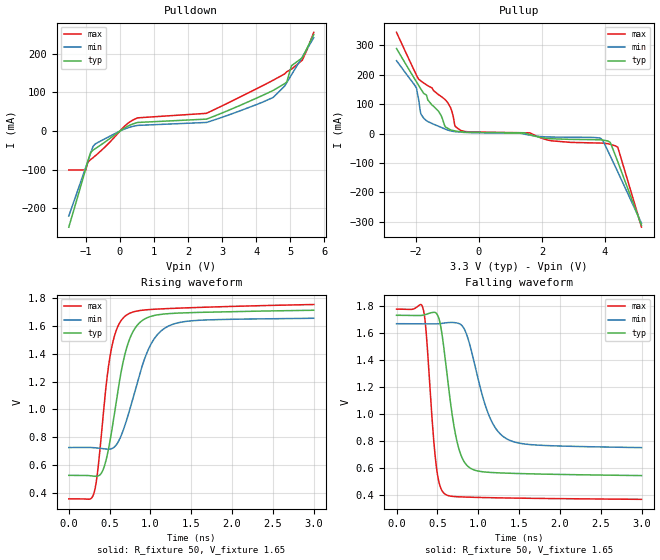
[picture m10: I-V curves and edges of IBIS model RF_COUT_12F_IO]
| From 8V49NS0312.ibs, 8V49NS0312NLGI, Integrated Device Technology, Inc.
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[Model]   RF_COUT_12F_IO
Model_type   Output
Polarity   Non-Inverting
|   typ   min   max
C_comp   2pF   1.5pF   2.5pF
Vmeas = 1.65V
Rref = 50
Cref = 0
Vref = 1.65V
|   typ   min   max
[Voltage range]   3.3V   3.135V   3.465V
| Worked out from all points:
|   slope of the pulldown table from 0 to 0.495 V, typ, clamps not added: 22.8 ohm
|   slope of the pullup table from 0 to 0.495 V, typ, clamps not added: 679 ohm
|   rising waveform, R_fixture 50, V_fixture 1.65: 20-80 % time 224ps typ, 305ps min, 167ps max; typ from 0.527 V to 1.71 V
|   falling waveform, R_fixture 50, V_fixture 1.65: 20-80 % time 167ps typ, 264ps min, 103ps max; typ from 1.73 V to 0.544 V
[Pulldown]
|Voltage   I (typ)   I (min)   I (max)
|Note, modeling breaks down at 250mA and above.  This is well beyond the functional   |
|operating range of the device.  Should this scenario occur, catastrophic failure and   |
|possible damage to the device and/or board is of higher concern than the I-V curve   |
|behavior.  The IBIS checker will flag currents in excess of 10A with warnings.  Lines   |
|with currents in excess of 0.35 A have been commented out.  The points still remain|
|available to the user if the user desires to use them.   |
|-3.30000e+00   -7.87257e-01   -6.73606e-01   -1.00473e-01
|-2.76540e+00   -6.25752e-01   -5.37099e-01   -1.00473e-01
|-2.74560e+00   -6.19818e-01   -5.32094e-01   -1.00473e-01
|-2.15160e+00   -4.42770e-01   -3.82988e-01   -1.00473e-01
|-1.97340e+00   -3.89863e-01   -3.38493e-01   -1.00473e-01
-1.498V   -248.5mA   -219.7mA   -100.5mA
-1V       -97.34mA   -93.55mA   -100.5mA
-943.8mV  -79.97mA   -79.2mA    -81.69mA
-787.2mV  -49.36mA   -39.79mA   -68.73mA
145.2mV   8.539mA    5.651mA    13.34mA
520mV     22.39mA    14.82mA    34.33mA
2.541V    31.09mA    22.47mA    46.04mA
4.462V    103.7mA    85.76mA    130mA
4.898V    127.4mA    125.6mA    153.7mA
5.034V    169.2mA    145.7mA    160.2mA
5.354V    190mA      192mA      183.8mA
5.689V    249.9mA    241.9mA    255.7mA
| 6.20400e+00   3.44362e-01   3.20728e-01   3.75765e-01
| 6.20480e+00   3.44511e-01   3.20853e-01   3.75955e-01
| 6.53920e+00   4.07706e-01   3.73926e-01   4.56273e-01
| 6.58480e+00   4.16452e-01   3.81302e-01   4.67382e-01
| 6.60000e+00   4.19374e-01   3.83769e-01   4.71095e-01
[Pullup]
|Voltage   I (typ)   I (min)   I (max)
|Note, modeling breaks down at 250mA and above.  This is well beyond the functional   |
|operating range of the device.  Should this scenario occur, catastrophic failure and   |
|possible damage to the device and/or board is of higher concern than the I-V curve   |
|behavior.  The IBIS checker will flag currents in excess of 10A with warnings.  Lines   |
|with currents in excess of 0.35 A have been commented out.  The points still remain|
|available to the user if the user desires to use them.   |
|-3.30000e+00   4.19294e-01   3.53041e-01   5.11558e-01
|-3.12180e+00   3.85262e-01   3.25457e-01   4.67756e-01
|-3.10200e+00   3.81510e-01   3.22421e-01   4.62928e-01
|-2.90400e+00   3.44298e-01   2.92352e-01   4.15047e-01
|-2.86440e+00   3.36919e-01   2.86398e-01   4.05555e-01
|-2.70600e+00   3.07607e-01   2.62761e-01   3.67856e-01
-2.607V   289.4mA    248.1mA    344.5mA
-1.973V   175.8mA    155.1mA    198.5mA
-1.835V   151.6mA    66.9mA     179.1mA
-1.736V   136.3mA    51.5mA     171.6mA
-1.063V   23.31mA    15.5mA     115.1mA
-884.4mV  12.55mA    9.074mA    85.79mA
-745.8mV  9.119mA    6.838mA    24.75mA
-567.6mV  6.452mA    5.027mA    10.81mA
3.848V    -20.97mA   -14.74mA   -31.9mA
4.165V    -29.65mA   -75.72mA   -36.12mA
4.402V    -95.36mA   -129.9mA   -45.91mA
5.155V    -312mA     -304.8mA   -317.9mA
| 5.29320e+00   -3.52204e-01   -3.37369e-01   -3.68931e-01
| 5.31300e+00   -3.57949e-01   -3.42027e-01   -3.76222e-01
| 5.41200e+00   -3.86685e-01   -3.65343e-01   -4.12676e-01
| 5.57040e+00   -4.32707e-01   -4.02726e-01   -4.71000e-01
| 5.66940e+00   -4.61500e-01   -4.26140e-01   -5.07454e-01
| 5.94660e+00   -5.42257e-01   -4.91910e-01   -6.09564e-01
| 5.98620e+00   -5.53812e-01   -5.01333e-01   -6.24160e-01
| 6.12480e+00   -5.94300e-01   -5.34374e-01   -6.75269e-01
| 6.14460e+00   -6.00090e-01   -5.39102e-01   -6.82574e-01
| 6.36240e+00   -6.63895e-01   -5.91253e-01   -7.63012e-01
| 6.38220e+00   -6.69707e-01   -5.96008e-01   -7.70333e-01
| 6.58020e+00   -7.27952e-01   -6.43704e-01   -8.43649e-01
| 6.60000e+00   -7.33790e-01   -6.48489e-01   -8.50992e-01
[Ramp]
|   typ   min   max
dV/dt_r   0.714/0.225n   0.563/0.307n   0.838/0.167n
dV/dt_f   0.727/0.169n   0.557/0.265n   0.867/0.105n
R_load =   50.0000
[Rising Waveform]
R_fixture = 50
V_fixture = 1.65   |Vcc_typ
V_fixture_min = 1.525  |Vcc_min
V_fixture_max = 1.7325 |Vcc_max
C_fixture = 0.0p
| Time   typ   min   max
0s        526.9mV    726.6mV    358.5mV
309.3ps   520.7mV    725.4mV    400.9mV
351.4ps   521.4mV    723.1mV    543.7mV
417.4ps   563mV      717.9mV    932.3mV
510.5ps   792.3mV    716mV      1.399V
693.7ps   1.41V      896.7mV    1.671V
804.8ps   1.576V     1.119V     1.702V
964ps     1.659V     1.416V     1.715V
1.201ns   1.686V     1.592V     1.723V
3ns       1.711V     1.654V     1.752V
[Falling Waveform]
R_fixture = 50
V_fixture = 1.65   |Vcc_typ
V_fixture_min = 1.55  |Vcc_min
V_fixture_max = 1.7325 |Vcc_max
C_fixture = 0.0p
| Time   typ   min   max
0s        1.733V     1.671V     1.779V
324.3ps   1.734V     1.67V      1.785V
363.4ps   1.74V      1.669V     1.607V
483.5ps   1.75V      1.669V     632.9mV
588.6ps   1.45V      1.676V     408.4mV
738.7ps   801.5mV    1.677V     386.8mV
903.9ps   598.7mV    1.5V       383mV
1.123ns   568.2mV    1.004V     379.8mV
1.342ns   561.7mV    818.8mV    377.4mV
3ns       543.8mV    751.3mV    367.4mV
